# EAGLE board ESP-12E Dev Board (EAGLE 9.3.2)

Size 70 x 75 mm. Coordinates in mm from the lower left corner, seen from the top.
Outline: 0,0 70,0 70,75 0,75 0,0
Copper layers (1*16): Top 0.035mm / dielectric 1.5mm / Bottom 0.035mm
Design rules "default *": minimum track width 6mil, minimum drill 0.35mm, track to track 6mil, track to pad 6mil, pad to pad 6mil, via to via 6mil, smd to smd 6mil, copper to edge 6mil, drill to drill 6mil, minimum pad ring 10mil, minimum via ring 8mil, stop-mask expansion 4mil, vias tented up to drill 0mil, thermal gap 10mil
Net classes: 0 default: width 0.203 mm; 1 power: width 0.762 mm

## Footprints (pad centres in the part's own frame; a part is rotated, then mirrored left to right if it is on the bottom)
C0805 = smd 1.3 x 1.5: 1 -0.95,0; 2 0.95,0
SMC_B = smd 1.6 x 2.4: + -1.5,0; - 1.5,0
UD-6,3X7,7_NICHICON = smd 2.8 x 1: + 2.35,0; - -2.35,0
SOD-123 = smd 1.397 x 1.397: + -1.651,0; - 1.651,0
ZX62B5PA33 = smd 0.4 x 1.35: D+ 0,1.95; D- -0.65,1.95; GND 1.3,1.95; ID 0.65,1.95; VCC -1.3,1.95 | smd 2.2 x 1.6: SHIELD_1 -3.15,1.825; SHIELD_6 3.15,1.825 | smd 1.8 x 1.9: SHIELD_2 -4,-0.725; SHIELD_5 4,-0.725 | smd 1.9 x 1.9: SHIELD_3 -1.2,-0.725; SHIELD_4 1.2,-0.725
5267-8 = drill 0.8 long: P$1 0,0; P$2 2.5,0; P$3 5,0; P$4 7.5,0; P$5 10,0; P$6 12.5,0; P$7 15,0; P$8 17.5,0
5267-4 = drill 0.8 long: P$1 0,0; P$2 2.5,0; P$3 5,0; P$4 7.5,0
5267-2 = drill 0.8 long: P$1 0,0; P$2 2.5,0
5267-3 = drill 0.8 long: P$1 0,0; P$2 2.5,0; P$3 5,0
POWER_JACK_SLOT = drill 1 pad 2 long: GND@1 2.5,1.39; GND@2 -2.5,-1.91; PWR 2.5,-4.91
CHIP-LED0805 = smd 1.2 x 1.2: A 0,-1.05; C 0,1.05
SOT65P210X100-6N = smd 1.1 x 0.4: 1 -0.9,0.65; 2 -0.9,0; 3 -0.9,-0.65; 4 0.9,-0.65; 5 0.9,0; 6 0.9,0.65
R0805 = smd 1.3 x 1.5: 1 -0.95,0; 2 0.95,0
TACTILE_SWITCH_SMD_6.0X3.5MM = smd 2.3 x 1.6: 1 -3.15,0; 2 3.15,0
ESP8266-ESP12E = smd 2 x 1.2: 1 -7.62,5.84; 2 -7.62,3.84; 3 -7.62,1.84; 4 -7.62,-0.16; 5 -7.62,-2.16; 6 -7.62,-4.16; 7 -7.62,-6.16; 8 -7.62,-8.16; 9 8.58,-8.16; 10 8.58,-6.16; 11 8.58,-4.16; 12 8.58,-2.16; 13 8.58,-0.16; 14 8.58,1.84; 15 8.58,3.84; 16 8.58,5.84 | smd 1.2 x 2: 17 -4.62,-10.16; 18 -2.62,-10.16; 19 -0.62,-10.16; 20 1.38,-10.16; 21 3.38,-10.16; 22 5.38,-10.16
SOT230P700X170-4N = smd 1.85 x 0.9: 1 -3.1,2.3; 2 -3.1,0; 3 -3.1,-2.3 | smd 1.85 x 3.2: 4 3.1,0
SOIC16 = smd 0.635 x 1.524: 1 -4.445,-2.695; 2 -3.175,-2.695; 3 -1.905,-2.695; 4 -0.635,-2.695; 5 0.635,-2.695; 6 1.905,-2.695; 7 3.175,-2.695; 8 4.445,-2.695; 9 4.445,2.695; 10 3.175,2.695; 11 1.905,2.695; 12 0.635,2.695; 13 -0.635,2.695; 14 -1.905,2.695; 15 -3.175,2.695; 16 -4.445,2.695
TSSOP14 = smd 0.305 x 0.991: 1 -1.95,-2.918; 2 -1.3,-2.918; 3 -0.65,-2.918; 4 0,-2.918; 5 0.65,-2.918; 6 1.3,-2.918; 7 1.95,-2.918; 8 1.95,2.918; 9 1.3,2.918; 10 0.65,2.918; 11 0,2.918; 12 -0.65,2.918; 13 -1.3,2.918; 14 -1.95,2.918
RK09K1130BGM = drill 1.2 pad 1.8: 1 -2.5,-12.5; 2 0,-12.5; 3 2.5,-12.5 | drill 2.97 pad 4.3: 4 4.3,-5.5; 5 -4.3,-5.5

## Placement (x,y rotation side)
C1  10uF  [C0805]  not placed on the board
C2  100nF  [C0805]  not placed on the board
C3  10uF  [C0805]  not placed on the board
C4  22uF  [C0805]  not placed on the board
C5  100uF  [SMC_B]  26.16,24.13 0 top
C6  220uF(optional)  [UD-6,3X7,7_NICHICON]  not placed on the board
C7  10uF  [C0805]  not placed on the board
C8  22uF  [C0805]  not placed on the board
C9  100nF  [C0805]  not placed on the board
C10  100nF  [C0805]  not placed on the board
C11  100uF  [SMC_B]  not placed on the board
C12  100nF  [C0805]  not placed on the board
D1  1N5819W  [SOD-123]  52.32,5.33 90 top
D2  1N5819W  [SOD-123]  34.29,8.64 90 top
J1  ZX62-B-5PA(33)  [ZX62B5PA33]  39.37,2.54 0 top
J2  LCD_CONN  [5267-8]  not placed on the board
J3  I2C  [5267-4]  not placed on the board
J4  LCD_BACKLIGHT  [5267-2]  not placed on the board
J5  I2C  [5267-4]  not placed on the board
J6  RADON_SENSOR  [5267-4]  not placed on the board
J8  ADC  [5267-3]  not placed on the board
J9  TEMP/HUM SENSOR  [5267-4]  not placed on the board
J10  BUTTON1  [5267-3]  not placed on the board
J11  DUST_SENSOR  [5267-4]  not placed on the board
JP1  POWER_JACKSLT  [POWER_JACK_SLOT]  61.98,6.1 270 top
LED1  green  [CHIP-LED0805]  not placed on the board
Q1  UMH3N  [SOT65P210X100-6N]  not placed on the board
R1  10k  [R0805]  not placed on the board
R2  10k  [R0805]  not placed on the board
R3  10k  [R0805]  not placed on the board
R4  10k  [R0805]  not placed on the board
R5  10k  [R0805]  not placed on the board
R6  470Ω  [R0805]  not placed on the board
R7  470Ω  [R0805]  not placed on the board
R8  470Ω  [R0805]  not placed on the board
R9  470Ω  [R0805]  not placed on the board
R10  470Ω  [R0805]  not placed on the board
R11  47k(1%)  [R0805]  not placed on the board
R12  10k(1%)  [R0805]  not placed on the board
R13  470Ω  [R0805]  not placed on the board
S1  RST  [TACTILE_SWITCH_SMD_6.0X3.5MM]  3.56,5.33 90 top
S2  FLASH  [TACTILE_SWITCH_SMD_6.0X3.5MM]  9.14,5.33 90 top
SJR1  ESP-12E  [ESP8266-ESP12E]  not placed on the board
U1  5V_REG  [SOT230P700X170-4N]  48.26,17.78 90 top
U2  3V3_REG  [SOT230P700X170-4N]  15.24,17.78 90 top
U3  CH340C  [SOIC16]  not placed on the board
U4  TXB0104  [TSSOP14]  not placed on the board
VR1  RK09K1130AAU(10k)  [RK09K1130BGM]  not placed on the board

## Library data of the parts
C1-C12 = rcl; SPICEPREFIX: C
D1 D2 = Seeed-Diode; MPN: SS0520-7-F
J1 = SamacSys_Parts; DESCRIPTION: USB Connectors MICRO B RECEPT RA SMT BTTM MNT; HEIGHT: 2.8mm; MANUFACTURER_NAME: Hirose; MANUFACTURER_PART_NUMBER: ZX62-B-5PA(33); MOUSER_PART_NUMBER: 798-ZX62-B-5PA33; MOUSER_PRICE-STOCK: https://www.mouser.com/Search/Refine.aspx?Keyword=798-ZX62-B-5PA33
J2-J6 J8-J11 = con-molex-spox
JP1 = kanflo
LED1 = adafruit
Q1 = SamacSys_Parts; DESCRIPTION: ROHM - UMH3NFHATN - TRANS, NPN, AUTO, 4.7K/4.7K, SOT-353; HEIGHT: 1mm; MANUFACTURER_NAME: ROHM Semiconductor; MANUFACTURER_PART_NUMBER: UMH3NFHATN; MOUSER_PART_NUMBER: 755-UMH3NFHATN; MOUSER_PRICE-STOCK: https://www.mouser.com/Search/Refine.aspx?Keyword=755-UMH3NFHATN
R1-R13 = rcl; SPICEPREFIX: R
S1 S2 = SparkFun-Switches; PROD_ID: SWCH-00815; SF_SKU: COM-08229
SJR1 = esp12e
U1 U2 = SamacSys_Parts; DESCRIPTION: 1A 5V LDO Linear Voltage Reg SOT-223 Diodes Inc AZ1117H-5.0TRE1, Single Linear Voltage Regulator, 1A 4.9 5.1 V, 1%, 3-Pin SOT-223; HEIGHT: 1.7mm; MANUFACTURER_NAME: Diodes Inc.; MANUFACTURER_PART_NUMBER: AZ1117H-5.0TRE1; MOUSER_PART_NUMBER: 621-AZ1117H-5.0TRE1; MOUSER_PRICE-STOCK: https://www.mouser.com/Search/Refine.aspx?Keyword=621-AZ1117H-5.0TRE1
U3 = ch340g
U4 = SparkFun-IC-Comms; PROD_ID: NA-XXXXX
VR1 = SamacSys_Parts; DESCRIPTION: Audio single pot. 10K Vertical 15mm,1B Alps RK09K Series, Linear Potentiometer with a 6 mm Dia. Shaft, 10k, +/-20%, Through Hole; HEIGHT: mm; MANUFACTURER_NAME: ALPS; MANUFACTURER_PART_NUMBER: RK09K1130A6S; MOUSER_PART_NUMBER: 688-RK09K1130A6S; MOUSER_PRICE-STOCK: https://www.mouser.com/Search/Refine.aspx?Keyword=688-RK09K1130A6S

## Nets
3.3V [power]: C8.2 C11.+ C12.2 J9.P$2 J10.P$2 R1.1 R2.1 R3.1 R4.1 R6.1 SJR1.8 U2.2 U2.4 U4.1 U4.8
5V [power]: C4.1 C5.+ C6.+ C7.1 C10.2 D2.- J2.P$2 J3.P$2 J5.P$2 J8.P$2 J11.P$2 U1.2 U1.4 U2.3 U3.16 U4.14 VR1.3
5V_INPUT [power]: D2.+ J1.VCC
12V [power]: C1.2 C3.1 D1.- J6.P$2 U1.3
12V_INPUT [power]: D1.+ JP1.PWR
ADC: R11.1 R12.2 SJR1.2
CS0_ESP: SJR1.17
D+_USB: J1.D+ U3.5
D-_USB: J1.D- U3.6
DTR: Q1.2 Q1.4 U3.13
EN: R3.2 SJR1.3
GND [power]: C1.1 C2.1 C3.2 C4.2 C5.- C6.- C7.2 C8.1 C9.1 C10.1 C11.- C12.1 J1.GND J1.SHIELD_1 J1.SHIELD_2 J1.SHIELD_3 J1.SHIELD_4 J1.SHIELD_5 J1.SHIELD_6 J2.P$1 J3.P$1 J4.P$1 J5.P$1 J6.P$1 J8.P$1 J9.P$1 J10.P$1 J11.P$1 JP1.GND@1 JP1.GND@2 LED1.C R5.1 R12.1 S1.2 S2.2 SJR1.9 U1.1 U2.1 U3.1 U4.7 VR1.1
GPIO0: Q1.3 R1.2 SJR1.12 U4.4
GPIO2: R2.2 SJR1.11 U4.5
GPIO4: J9.P$4 SJR1.13 U4.3
GPIO5: J9.P$3 SJR1.14 U4.2
GPIO9: SJR1.19
GPIO10: SJR1.20
GPIO12: R10.1 SJR1.6
GPIO13: J6.P$4 SJR1.7
GPIO14: R13.1 SJR1.5
GPIO15: J10.P$3 R5.2 SJR1.10
GPIO16: J11.P$4 R8.1 SJR1.4
LED+_5V: J2.P$7 J4.P$2 U4.11
LED-_5V: J2.P$8 U4.10
MISO_ESP: SJR1.18
MOSI_ESP: SJR1.21
N$1: C9.2 U3.4
N$2: J2.P$3 VR1.2
N$3: R9.2 U3.2
N$4: LED1.A R6.2
N$5: J8.P$3 R11.2
N$6: J6.P$3 R10.2
N$9: J11.P$3 R13.2
POWER: R7.2 S1.1
POWER1: R8.2 S2.1
RST: C2.2 Q1.6 R4.2 R7.1 SJR1.1
RTS: Q1.1 Q1.5 U3.14
RXD: R9.1 SJR1.15
SCL_5V: J2.P$4 J3.P$3 J5.P$3 U4.13
SCLK_ESP: SJR1.22
SDA_5V: J2.P$5 J3.P$4 J5.P$4 U4.12
TXD: SJR1.16 U3.3

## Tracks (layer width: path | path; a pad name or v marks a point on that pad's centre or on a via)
3.3V  (14 unrouted)
5V  (16 unrouted)
5V_INPUT  (1 unrouted)
12V  (4 unrouted)
12V_INPUT  (1 unrouted)
ADC  (2 unrouted)
D+_USB  (1 unrouted)
D-_USB  (1 unrouted)
DTR  (2 unrouted)
EN  (1 unrouted)
GND  (40 unrouted)
GPIO0  (3 unrouted)
GPIO2  (2 unrouted)
GPIO4  (2 unrouted)
GPIO5  (2 unrouted)
GPIO12  (1 unrouted)
GPIO13  (1 unrouted)
GPIO14  (1 unrouted)
GPIO15  (2 unrouted)
GPIO16  (2 unrouted)
LED+_5V  (2 unrouted)
LED-_5V  (1 unrouted)
N$1  (1 unrouted)
N$2  (1 unrouted)
N$3  (1 unrouted)
N$4  (1 unrouted)
N$5  (1 unrouted)
N$6  (1 unrouted)
N$9  (1 unrouted)
POWER  (1 unrouted)
POWER1  (1 unrouted)
RST  (4 unrouted)
RTS  (2 unrouted)
RXD  (1 unrouted)
SCL_5V  (3 unrouted)
SDA_5V  (3 unrouted)
TXD  (1 unrouted)

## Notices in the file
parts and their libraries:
SparkFun-Switches: Licensing: Creative Commons ShareAlike 4.0 International - https://creativecommons.org/licenses/by-sa/4.0
